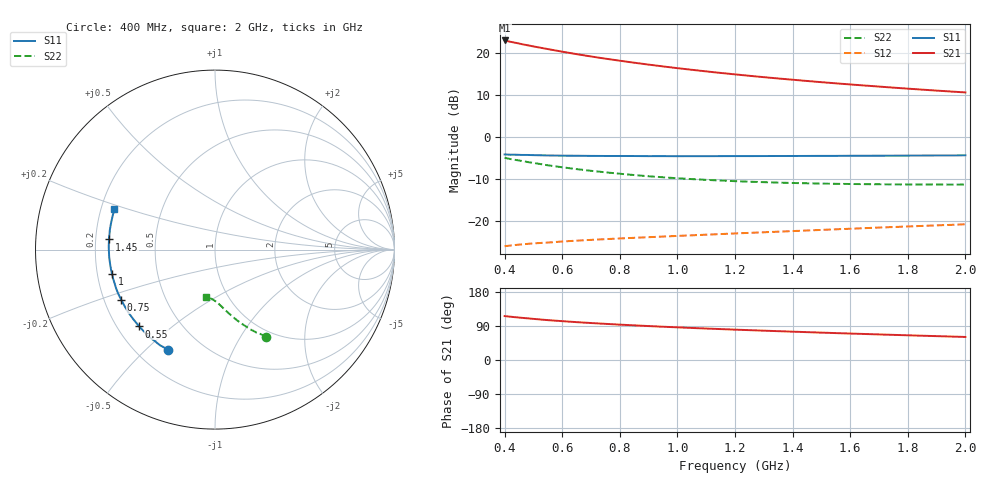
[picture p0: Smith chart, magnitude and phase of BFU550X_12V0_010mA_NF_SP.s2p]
! Filename:  P:\Prog\Test\Noise\ATS_data\Testdata_Net\BFU550X no attenuator noise\BFU550X_APG2013_44_C05_12p0V_010mA_NF_CM01_D.sf
! Date/Time: Fri 26/Jul/2013 14:37:14
! BFU550X_APG2013_44_C05_12p0V_1to10mA_NF_CM01_Bias5_R.sf
! Noise Parameter Data File
! BFU550X_APG2013_44_C05_12p0V_1to10mA_NF_CM01
! Date/time: Thu Jul 25 09:36:35 2013
! VAR V_out= 12.001000
! VAR I_out= 9.995000
! VAR V_in= 0.795000
! VAR I_in= 0.094505
! Device data file deembeded for feedlines and parallel
! Original file: \BFU550X no attenuator noise\BFU550X_APG2013_44_C05_12p0V_010mA_NF_CM01_R.sf
! Feed-files: PR005V01_100713_Feed1.s2p, PR005V01_100713_Feed2.s2p
! Parallel-file: PR005V01_100713_Par.s2p
# MHz S MA R 50
!  Freq-MHz  S11-mag  S11-arg  S21-mag  S21-arg  S12-mag  S12-arg  S22-mag  S22-arg
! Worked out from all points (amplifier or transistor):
!   37 points, 400 MHz to 2 GHz, reference 50 ohm
!   highest |S21| = 23.1 dB at 400 MHz (marker M1)
!   |S21| within 3 dB of that: start of sweep to 626.8 MHz
!   unconditionally stable (mu >= 1): nowhere
!   at 500 MHz: K = 0.41, MSG = 23.6 dB, |S12| = -25.5 dB
!   at 1.1 GHz: K = 0.75, MSG = 19.5 dB, |S12| = -23.4 dB
!   at 2 GHz: K = 1.00, MSG = 15.8 dB, |S12| = -20.9 dB
!   lowest NFmin = 0.83 dB at 440 MHz
!   S11 on the Smith chart (normalised r, x): 400 MHz: 0.32, -0.59; 550 MHz: 0.29, -0.39; 750 MHz: 0.27, -0.23; 1 GHz: 0.26, -0.11; 1.45 GHz: 0.26, +0.04; 2 GHz: 0.26, +0.18
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400  0.6182 -115.0  14.29 115.8  0.04941 44.0  0.5625 -59.4
420  0.6142 -117.9  13.78 114.3  0.05029 43.4  0.5449 -60.9
440  0.6132 -120.9  13.35 112.7  0.05117 42.7  0.5302 -62.0
460  0.6099 -123.4  12.9 111.3  0.05192 42.0  0.5169 -63.5
500  0.6067 -128.7  12.12 108.5  0.05335 40.9  0.4902 -65.8
550  0.6014 -134.7  11.27 105.2  0.0546 40.1  0.4583 -68.3
600  0.598 -139.5  10.49 102.5  0.05617 39.4  0.4343 -70.6
650  0.5964 -144.0  9.8 99.9  0.05751 38.9  0.4128 -72.7
700  0.5939 -148.2  9.193 97.5  0.05875 38.6  0.3937 -74.5
750  0.5928 -151.8  8.653 95.4  0.05998 38.4  0.3778 -76.1
800  0.5925 -155.3  8.175 93.3  0.06113 38.3  0.3634 -77.8
850  0.5919 -158.5  7.74 91.4  0.0622 38.2  0.3504 -79.3
950  0.5904 -164.3  6.988 87.8  0.06442 38.5  0.3296 -82.0
1000  0.5892 -166.9  6.661 86.2  0.0655 38.7  0.3209 -83.1
1100  0.5898 -171.7  6.091 83.0  0.0678 39.1  0.307 -85.4
1200  0.591 -176.0  5.612 80.1  0.07014 39.6  0.2962 -87.5
1300  0.5916 -179.9  5.199 77.4  0.07248 40.1  0.2881 -89.4
1450  0.5934 174.5  4.681 73.5  0.07611 40.8  0.2793 -92.2
1500  0.5943 172.8  4.526 72.2  0.0773 41.1  0.2769 -93.1
1600  0.596 169.5  4.253 69.8  0.07986 41.5  0.274 -94.8
1750  0.598 165.0  3.895 66.3  0.08367 42.1  0.2709 -97.3
2000  0.6035 158.1  3.414 60.8  0.09038 43.0  0.2699 -101.2
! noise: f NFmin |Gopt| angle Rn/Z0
400  0.8518  0.05938  156  0.1003
460  0.8482  0.09893  169.9  0.0807
600  0.9051  0.08491  155.1  0.0919
800  0.8946  0.153  159.3  0.075
1000  0.9206  0.1788  161.5  0.0729
1200  0.9297  0.2188  168.3  0.0691
1400  0.9747  0.2539  172.4  0.0626
1600  1.006  0.2728  178.4  0.0636
1800  1.023  0.3108  -178.8  0.0592
2000  1.043  0.3296  -174.3  0.0633
